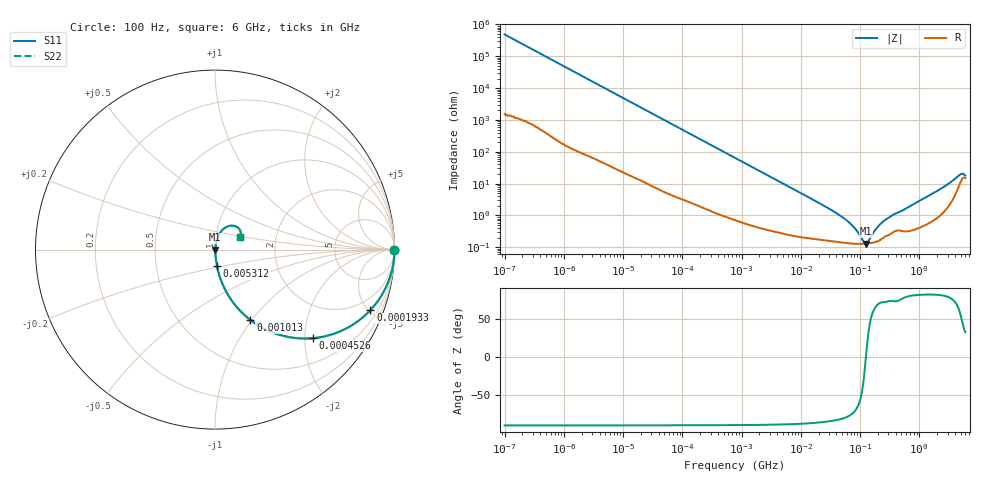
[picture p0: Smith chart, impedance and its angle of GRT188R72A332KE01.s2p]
!Murata Part Number: GRT188R72A332KE01
!These Parameters are Measured in Series Mode Connection
!Data Generated on Jun 19, 2026
!  o--ll--o
!Port1  Port2
!  o------o
!Operation Temp=25[degC], DC Bias Voltage=0[V]
!Freq. Start=100[Hz] Stop=6[GHz] 401[Steps]
# Hz S RI R 50
!Freq.(Hz) S11(Real) S11(Imag) S21(Real) S21(Imag) S12(Real) S12(Imag) S22(Real) S22(Imag)
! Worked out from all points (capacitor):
!   401 points, 100 Hz to 6 GHz, reference 50 ohm
!   read as one part in series: C = 3.29 nF near 109 Hz
!   lowest |Z| = 131 mohm at 127.6 MHz (marker M1)
!   series resonance near 125.6 MHz, so ESL is about 490 pH
!   S11 on the Smith chart (normalised r, x): 100 Hz: open; 193.3 kHz: 1.04, -5.11; 452.6 kHz: 1.02, -2.19; 1.013 MHz: 1.01, -0.98; 5.312 MHz: 1.01, -0.19; 6 GHz: 1.30, +0.19
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100  1 -0.000207  7e-07 0.000207  7e-07 0.000207  1 -0.000207
2008  1 -0.00412  3.23e-05 0.00412  3.23e-05 0.00412  1 -0.00412
40335  0.9929 -0.0815  0.00712 0.0815  0.00712 0.0815  0.9929 -0.0815
103284  0.9567 -0.2003  0.0433 0.2003  0.0433 0.2003  0.9567 -0.2003
193316  0.8654 -0.3376  0.1346 0.3376  0.1346 0.3376  0.8654 -0.3376
452617  0.5452 -0.4933  0.4548 0.4933  0.4548 0.4933  0.5452 -0.4933
774597  0.294 -0.4501  0.706 0.4501  0.706 0.4501  0.294 -0.4501
1013323  0.1975 -0.3921  0.8025 0.3921  0.8025 0.3921  0.1975 -0.3921
1983483  0.0631 -0.2352  0.9369 0.2352  0.9369 0.2352  0.0631 -0.2352
5311619  0.0114 -0.0934  0.9886 0.0934  0.9886 0.0934  0.0114 -0.0934
1.555665e7  0.00289 -0.0321  0.9971 0.0321  0.9971 0.0321  0.00289 -0.0321
3.64232e7  0.00169 -0.013  0.9983 0.013  0.9983 0.013  0.00169 -0.013
5.960426e7  0.0014 -0.00682  0.9986 0.00682  0.9986 0.00682  0.0014 -0.00682
8.154455e7  0.0013 -0.00375  0.9987 0.00375  0.9987 0.00375  0.0013 -0.00375
1.166697e8  0.00129 -0.000624  0.9987 0.000624  0.9987 0.000624  0.00129 -0.000624
1.275994e8  0.0013 0.000135  0.9987 -0.000135  0.9987 -0.000135  0.0013 0.000135
2.088084e8  0.00164 0.00454  0.9984 -0.00454  0.9984 -0.00454  0.00164 0.00454
3.124326e8  0.00254 0.00844  0.9975 -0.00844  0.9975 -0.00844  0.00254 0.00844
2.450438e9  0.0165 0.071  0.9835 -0.071  0.9835 -0.071  0.0165 0.071
4.586474e9  0.0912 0.1337  0.9088 -0.1337  0.9088 -0.1337  0.0912 0.1337
5.245841e9  0.1352 0.1156  0.8648 -0.1156  0.8648 -0.1156  0.1352 0.1156
6e9  0.1365 0.0723  0.8635 -0.0723  0.8635 -0.0723  0.1365 0.0723
